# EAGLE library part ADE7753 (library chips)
Single-Phase Multifunction Metering IC
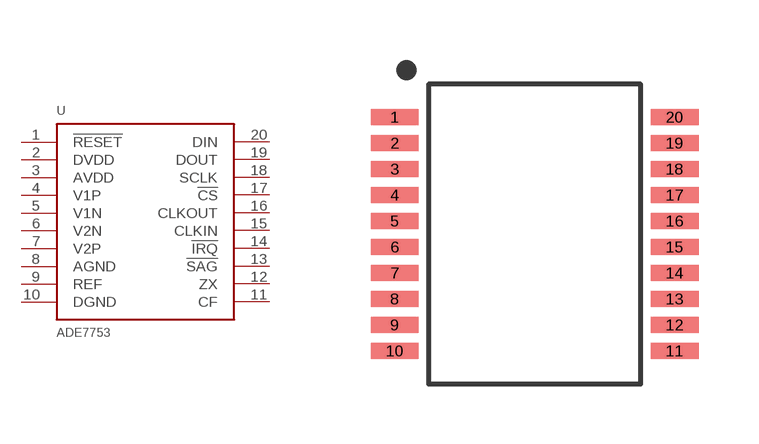
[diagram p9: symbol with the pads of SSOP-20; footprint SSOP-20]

Designator prefix U

## ADE7753ARS (DIGIKEY: ADE7753ARSZRLCT-ND; MOUSER: 584-ADE7753ARSZR; NEWARK: 59K0984)  [SSOP-20]
1  !RESET
2  DVDD
3  AVDD
4  V1P
5  V1N
6  V2N
7  V2P
8  AGND
9  REF
10  DGND
11  CF
12  ZX
13  !SAG
14  !IRQ
15  CLKIN
16  CLKOUT
17  !CS
18  SCLK
19  DOUT
20  DIN

## Footprint SSOP-20 (pad centres in mm)
smd 1.2 x 0.4: 1 -3.5,2.925; 2 -3.5,2.275; 3 -3.5,1.625; 4 -3.5,0.975; 5 -3.5,0.325; 6 -3.5,-0.325; 7 -3.5,-0.975; 8 -3.5,-1.625; 9 -3.5,-2.275; 10 -3.5,-2.925; 11 3.5,-2.925; 12 3.5,-2.275; 13 3.5,-1.625; 14 3.5,-0.975; 15 3.5,-0.325; 16 3.5,0.325; 17 3.5,0.975; 18 3.5,1.625; 19 3.5,2.275; 20 3.5,2.925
